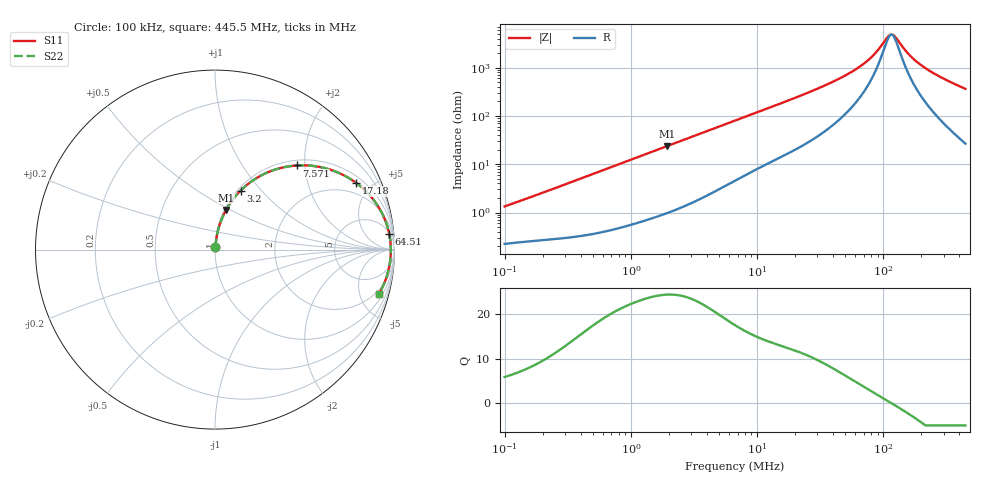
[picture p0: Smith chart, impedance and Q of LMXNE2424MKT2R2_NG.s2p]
! LMXNE2424MKT2R2_NG  S-PARAMETER MODEL  ( General Type )
! Model Generated by TAIYO YUDEN Corporation (https://www.yuden.co.jp/en/)
! Version 1.0
! TAIYO YUDEN Control No. 191023NI43SB-FBB
! Copyright(c) 2019 TAIYO YUDEN CO.,LTD. All Rights Reserved.
! Product Description (link to TY-COMPAS)
! https://ds.yuden.co.jp/TYCOMPAS/or/detail?pn=LMXNE2424MKT2R2MNG&u=M
! Products Name : Inductors
! Characteristics :
!  Inductance : 2.2 uH , SRF(min) : 72 MHz , DC Resistance(max) : 0.168 Ohm
!  Rated Current : Saturation :1700 mA , Temp Rise : 1000 mA (40 degC)
!  Case Size : 2.4 x 2.4 / 0.095 x 0.095 [mm/inch] , Thickness : 1.2 / 0.047 [mm/inch]
!  (Conditions: Temperature = 25 degC , DC Bias Current/Voltage = 0A / 0V)
! External Node Assignments :
!  1  o---GGG---o  2
! GND o---------o GND
! Frequency Range : 0.1MHz  -  445.549718MHz  [ 402 STEP ]
# MHz S RI R 50
! Freq[MHz].  S11 Real  S11 Imag  S21 Real  S21 Imag  S12 Real  S12 Imag  S22 Real  S22 Imag
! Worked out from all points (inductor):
!   401 points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, 100 kHz to 445.5 MHz, reference 50 ohm
!   read as one part in series: L = 2.07 uH near 104.3 kHz
!   highest Q = 24.4 at 1.933 MHz (marker M1), where L = 1.95 uH
!   self-resonance near 115.7 MHz
!   S11 on the Smith chart (normalised r, x): 100 kHz: 1.00, +0.03; 3.2 MHz: 1.03, +0.78; 7.571 MHz: 1.11, +1.81; 17.18 MHz: 1.32, +4.05; 64.51 MHz: 6, +20; 445.5 MHz: 1.53, -7.26
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0.1  0.00241 0.0131  0.9976 -0.0131  0.9976 -0.0131  0.00241 0.0131
0.408498  0.00588 0.0509  0.9941 -0.0509  0.9941 -0.0509  0.00588 0.0509
0.870143  0.0164 0.1058  0.9836 -0.1058  0.9836 -0.1058  0.0164 0.1058
1.668708  0.0478 0.1937  0.9522 -0.1937  0.9522 -0.1937  0.0478 0.1937
1.933018  0.0614 0.2204  0.9386 -0.2204  0.9386 -0.2204  0.0614 0.2204
3.200145  0.1424 0.3285  0.8576 -0.3285  0.8576 -0.3285  0.1424 0.3285
4.57349  0.2453 0.4067  0.7547 -0.4067  0.7547 -0.4067  0.2453 0.4067
6.81664  0.4066 0.4633  0.5934 -0.4633  0.5934 -0.4633  0.4066 0.4633
7.571493  0.4542 0.4687  0.5458 -0.4687  0.5458 -0.4687  0.4542 0.4687
11.0505  0.6241 0.4508  0.3759 -0.4508  0.3759 -0.4508  0.6241 0.4508
17.17706  0.7867 0.3715  0.2133 -0.3715  0.2133 -0.3715  0.7867 0.3715
27.26705  0.8942 0.2627  0.1058 -0.2627  0.1058 -0.2627  0.8942 0.2627
44.20279  0.9504 0.1577  0.0496 -0.1577  0.0496 -0.1577  0.9504 0.1577
64.51342  0.9703 0.0894  0.0297 -0.0894  0.0297 -0.0894  0.9703 0.0894
83.00742  0.9768 0.0494  0.0232 -0.0494  0.0232 -0.0494  0.9768 0.0494
111.3854  0.9797 0.00561  0.0203 -0.00561  0.0203 -0.00561  0.9797 0.00561
116.1643  0.9798 -0.000543  0.0202 0.000543  0.0202 0.000543  0.9798 -0.000543
123.7199  0.9798 -0.00978  0.0202 0.00978  0.0202 0.00978  0.9798 -0.00978
159.1866  0.9778 -0.0474  0.0222 0.0474  0.0222 0.0474  0.9778 -0.0474
209.1681  0.9716 -0.0912  0.0284 0.0912  0.0284 0.0912  0.9716 -0.0912
292.7193  0.9559 -0.1526  0.0441 0.1526  0.0441 0.1526  0.9559 -0.1526
445.5497  0.9143 -0.2456  0.0857 0.2456  0.0857 0.2456  0.9143 -0.2456
